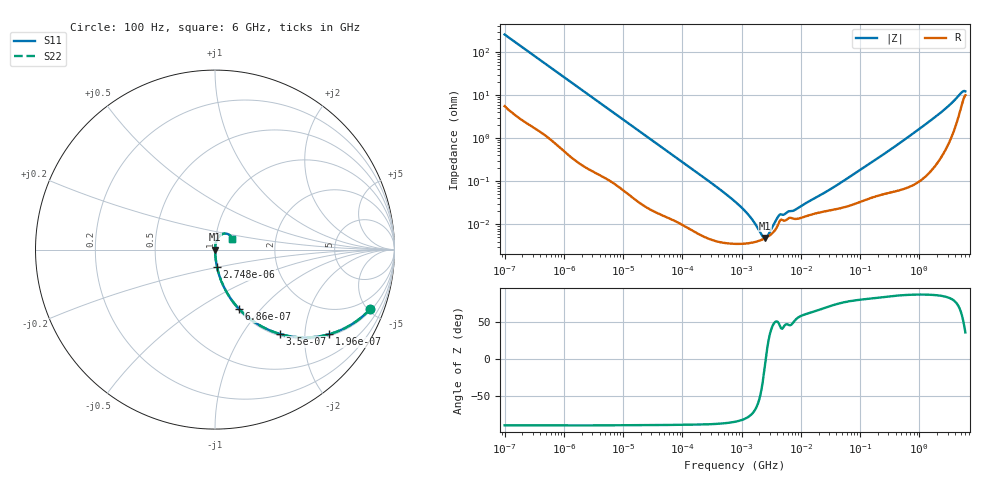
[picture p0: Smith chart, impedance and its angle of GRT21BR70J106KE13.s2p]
!Murata Part Number: GRT21BR70J106KE13
!These Parameters are Measured in Series Mode Connection
!Data Generated on Jun 19, 2026
!  o--ll--o
!Port1  Port2
!  o------o
!Operation Temp=25[degC], DC Bias Voltage=0[V]
!Freq. Start=100[Hz] Stop=6[GHz] 401[Steps]
# Hz S RI R 50
!Freq.(Hz) S11(Real) S11(Imag) S21(Real) S21(Imag) S12(Real) S12(Imag) S22(Real) S22(Imag)
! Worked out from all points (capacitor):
!   401 points, 100 Hz to 6 GHz, reference 50 ohm
!   read as one part in series: C = 6.15 uF near 109 Hz
!   lowest |Z| = 4.81 mohm at 2.481 MHz (marker M1)
!   series resonance near 2.559 MHz, so ESL is about 630 pH
!   S11 on the Smith chart (normalised r, x): 100 Hz: 1.11, -5.16; 196 Hz: 1.05, -2.65; 350 Hz: 1.03, -1.49; 686 Hz: 1.02, -0.77; 2.748 kHz: 1.00, -0.20; 6 GHz: 1.20, +0.14
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100  0.8642 -0.3319  0.1358 0.3319  0.1358 0.3319  0.8642 -0.3319
196  0.6353 -0.4714  0.3647 0.4714  0.3647 0.4714  0.6353 -0.4714
350  0.361 -0.4698  0.639 0.4698  0.639 0.4698  0.361 -0.4698
686  0.1346 -0.3311  0.8654 0.3311  0.8654 0.3311  0.1346 -0.3311
2008  0.0197 -0.1302  0.9803 0.1302  0.9803 0.1302  0.0197 -0.1302
2748  0.0112 -0.0963  0.9888 0.0963  0.9888 0.0963  0.0112 -0.0963
8047  0.00192 -0.0337  0.9981 0.0337  0.9981 0.0337  0.00192 -0.0337
40335  0.000223 -0.00688  0.9998 0.00688  0.9998 0.00688  0.000223 -0.00688
774597  3.54e-05 -0.000338  1 0.000338  1 0.000338  3.54e-05 -0.000338
1159002  3.59e-05 -0.000198  1 0.000198  1 0.000198  3.59e-05 -0.000198
1734173  3.94e-05 -9.01e-05  1 9.01e-05  1 9.01e-05  3.94e-05 -9.01e-05
2481164  4.76e-05 -7e-06  1 7e-06  1 7e-06  4.76e-05 -7e-06
3394479  6.48e-05 6.66e-05  0.9999 -6.66e-05  0.9999 -6.66e-05  6.48e-05 6.66e-05
4440638  0.000121 0.000119  0.9999 -0.000119  0.9999 -0.000119  0.000121 0.000119
7947587  0.000134 0.00017  0.9999 -0.00017  0.9999 -0.00017  0.000134 0.00017
1.555665e7  0.000171 0.000336  0.9998 -0.000336  0.9998 -0.000336  0.000171 0.000336
4.165952e7  0.00023 0.000801  0.9998 -0.000801  0.9998 -0.000801  0.00023 0.000801
3.124326e8  0.00057 0.00522  0.9994 -0.00522  0.9994 -0.00522  0.00057 0.00522
1.369159e9  0.00193 0.0227  0.9981 -0.0227  0.9981 -0.0227  0.00193 0.0227
3.205649e9  0.0113 0.0568  0.9887 -0.0568  0.9887 -0.0568  0.0113 0.0568
5.016141e9  0.0553 0.0896  0.9447 -0.0896  0.9447 -0.0896  0.0553 0.0896
6e9  0.0948 0.0592  0.9052 -0.0592  0.9052 -0.0592  0.0948 0.0592
